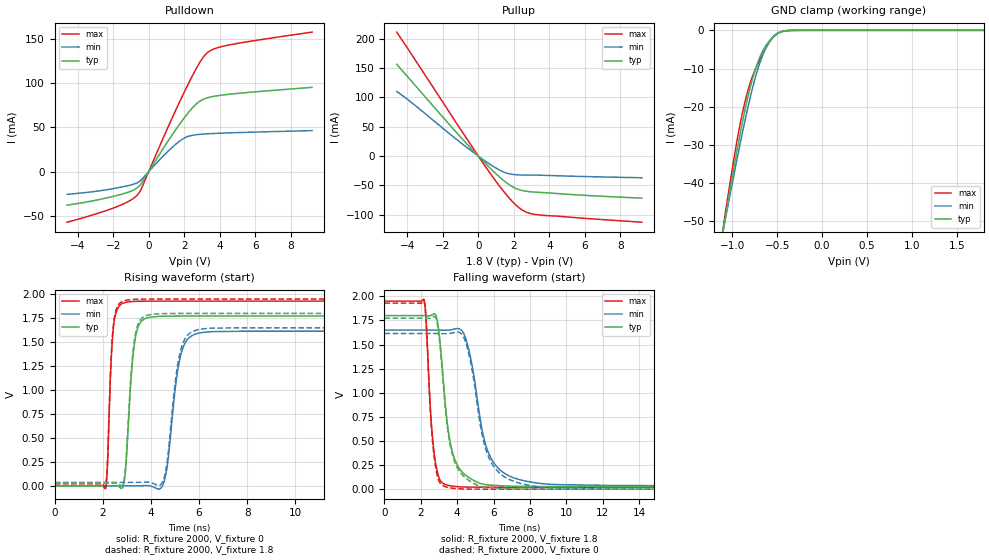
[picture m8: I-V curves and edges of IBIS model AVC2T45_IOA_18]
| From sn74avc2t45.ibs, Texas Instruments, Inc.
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[Model]   AVC2T45_IOA_18
Model_type  I/O
Vinl=0.5775
Vinh=1.2675
Enable   Active-Low
Vref =   0
Rref =   2000
Cref =   15p
Vmeas =   0.9
| variable   typ   min   max
C_comp   5.13pF   4.43pF   5.79pF
| C_pullup   4.65pF   3.47pF   6.78pF
| C_pulldown   4.55pF   4.02pF   4.94pF
| C_tri-state   5.13pF   4.43pF   5.79pF
[Temperature Range]   40   100   -40
| Ambient temperature   25   85   -40
[Voltage range]   1.8   1.65   1.95
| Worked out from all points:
|   slope of the pulldown table from 0 to 0.27 V, typ, clamps not added: 30.8 ohm
|   slope of the pullup table from 0 to 0.27 V, typ, clamps not added: 31.4 ohm
|   GND clamp passes 1 mA (typ) near -0.50 V on its own axis
|   rising waveform, R_fixture 2000, V_fixture 0: 20-80 % time 283ps typ, 440ps min, 184ps max; typ from 0 V to 1.77 V
|   falling waveform, R_fixture 2000, V_fixture 1.8: 20-80 % time 647ps typ, 989ps min, 371ps max; typ from 1.8 V to 0.027 V
|   rising waveform, R_fixture 2000, V_fixture 1.8: 20-80 % time 281ps typ, 432ps min, 183ps max; typ from 0.027 V to 1.8 V
|   falling waveform, R_fixture 2000, V_fixture 0: 20-80 % time 649ps typ, 989ps min, 359ps max; typ from 1.77 V to 0 V
[GND Clamp]
| AVC2T45_IOA_18
|   Voltage   I(typ)   I(min)   I(max)
-4.6V     -597.8mA   -546.6mA   -662.5mA
-1.1V     -52.11mA   -52.52mA   -51.59mA
-1.075V   -48.66mA   -49.4mA    -47.7mA
-930mV    -29.5mA    -31.88mA   -26.82mA
-830mV    -17.94mA   -20.74mA   -16.24mA
-755mV    -11.24mA   -13.46mA   -10.89mA
-675mV    -6.119mA   -7.407mA   -6.788mA
-595mV    -3.054mA   -3.247mA   -3.436mA
-520mV    -1.318mA   -1.132mA   -1.268mA
-445mV    -373.4uA   -312uA     -266.4uA
-300mV    -9.535uA   -12.09uA   -2.471uA
1.8V      910.1pA    145.3nA    97.77pA
[Pulldown]
| AVC2T45_IOA_18
|   Voltage   I(typ)   I(min)   I(max)
-4.6V     -37.94mA   -25.73mA   -57.23mA
-1.805V   -27.11mA   -18.54mA   -39.83mA
-1.045V   -22.5mA    -15.36mA   -32.7mA
-590mV    -17.44mA   -12.06mA   -25.35mA
-395mV    -12.81mA   -8.801mA   -18.52mA
1.005V    31.93mA    21.31mA    46.48mA
1.825V    55.97mA    35.61mA    82.46mA
2.68V     76.51mA    41.68mA    116.5mA
3.045V    81.48mA    42.38mA    128.6mA
3.34V     83.6mA     42.77mA    135mA
4.58V     87.53mA    43.81mA    143.4mA
9.2V      95.24mA    46.32mA    157.7mA
[Pullup]
| AVC2T45_IOA_18
|   Voltage   I(typ)   I(min)   I(max)
-4.6V     156.3mA    109.9mA    211.2mA
-3.695V   125.1mA    89.45mA    169.9mA
-1.245V   40.55mA    28.8mA     56.51mA
535mV     -16.77mA   -11.6mA    -23.84mA
1.065V    -32.16mA   -21.66mA   -46.14mA
1.49V     -43.16mA   -27.88mA   -62.67mA
1.925V    -52.28mA   -31.05mA   -77.72mA
2.305V    -57.27mA   -32.09mA   -88.3mA
2.77V     -60.1mA    -32.26mA   -96.25mA
3.4V      -61.74mA   -32.39mA   -100.1mA
9.2V      -71.58mA   -36.85mA   -112.5mA
[Ramp]
| AVC2T45_IOA_18
| variable   typ   min   max
dV/dt_r   1.08/3.00E-10   0.99/4.54E-10   1.18/1.95E-10
dV/dt_f   1.08/6.52E-10   0.98/9.96E-10   1.17/3.75E-10
R_load = 2000
[Rising Waveform]
| AVC2T45_IOA_18
R_fixture =   2000
C_fixture =   0
L_fixture =   0
V_fixture =   0
V_fixture_min = 0
V_fixture_max = 0
|   Time   V(typ)   V(min)   V(max)
0s        21.36nV    98.35nV    643.8pV
2.11ns    38.81uV    19.13nV    -31.01mV
2.445ns   905.4uV    -19.99uV   1.669V
2.97ns    253.3mV    6.678uV    1.917V
3.32ns    1.495V     -166.1uV   1.925V
3.91ns    1.758V     2.004mV    1.928V
4.535ns   1.77V      36.17mV    1.929V
5.225ns   1.772V     1.352V     1.929V
6.02ns    1.772V     1.596V     1.929V
34.99ns   1.772V     1.614V     1.929V
[Falling Waveform]
| AVC2T45_IOA_18
R_fixture =   2000
C_fixture =   0
L_fixture =   0
V_fixture =   1.8
V_fixture_min = 1.65
V_fixture_max = 1.95
|   Time   V(typ)   V(min)   V(max)
0s        1.8V       1.65V      1.95V
2.175ns   1.8V       1.65V      1.965V
2.725ns   1.819V     1.65V      387.9mV
2.99ns    1.638V     1.649V     124.6mV
3.405ns   767.2mV    1.648V     44.88mV
3.76ns    369.3mV    1.657V     31.29mV
4.31ns    171.1mV    1.63V      23.02mV
5.69ns    44.91mV    393.1mV    20.54mV
7.415ns   29.02mV    99.5mV     20.46mV
34.99ns   27.15mV    36.2mV     20.45mV
[Rising Waveform]
| AVC2T45_IOA_18
R_fixture =   2000
C_fixture =   0
L_fixture =   0
V_fixture =   1.8
V_fixture_min = 1.65
V_fixture_max = 1.95
|   Time   V(typ)   V(min)   V(max)
0s        27.15mV    36.2mV     20.45mV
2.11ns    27.19mV    36.2mV     -10.37mV
2.445ns   28.05mV    36.19mV    1.694V
2.965ns   270.3mV    36.21mV    1.938V
3.32ns    1.533V     36.04mV    1.947V
3.94ns    1.786V     37.08mV    1.95V
4.53ns    1.798V     73.29mV    1.95V
5.205ns   1.8V       1.387V     1.95V
6ns       1.8V       1.633V     1.95V
34.99ns   1.8V       1.65V      1.95V
[Falling Waveform]
| AVC2T45_IOA_18
R_fixture =   2000
C_fixture =   0
L_fixture =   0
V_fixture =   0
V_fixture_min = 0
V_fixture_max = 0
|   Time   V(typ)   V(min)   V(max)
0s        1.772V     1.614V     1.929V
2.175ns   1.772V     1.614V     1.944V
2.725ns   1.791V     1.615V     346.3mV
2.985ns   1.616V     1.614V     92.81mV
3.39ns    762.5mV    1.613V     23.19mV
3.755ns   345.8mV    1.621V     9.656mV
4.32ns    141.6mV    1.588V     2.129mV
5.68ns    17.04mV    356.6mV    83.1uV
7.45ns    1.542mV    60.71mV    9.245uV
34.99ns   88.37nV    464.3nV    160.5nV
